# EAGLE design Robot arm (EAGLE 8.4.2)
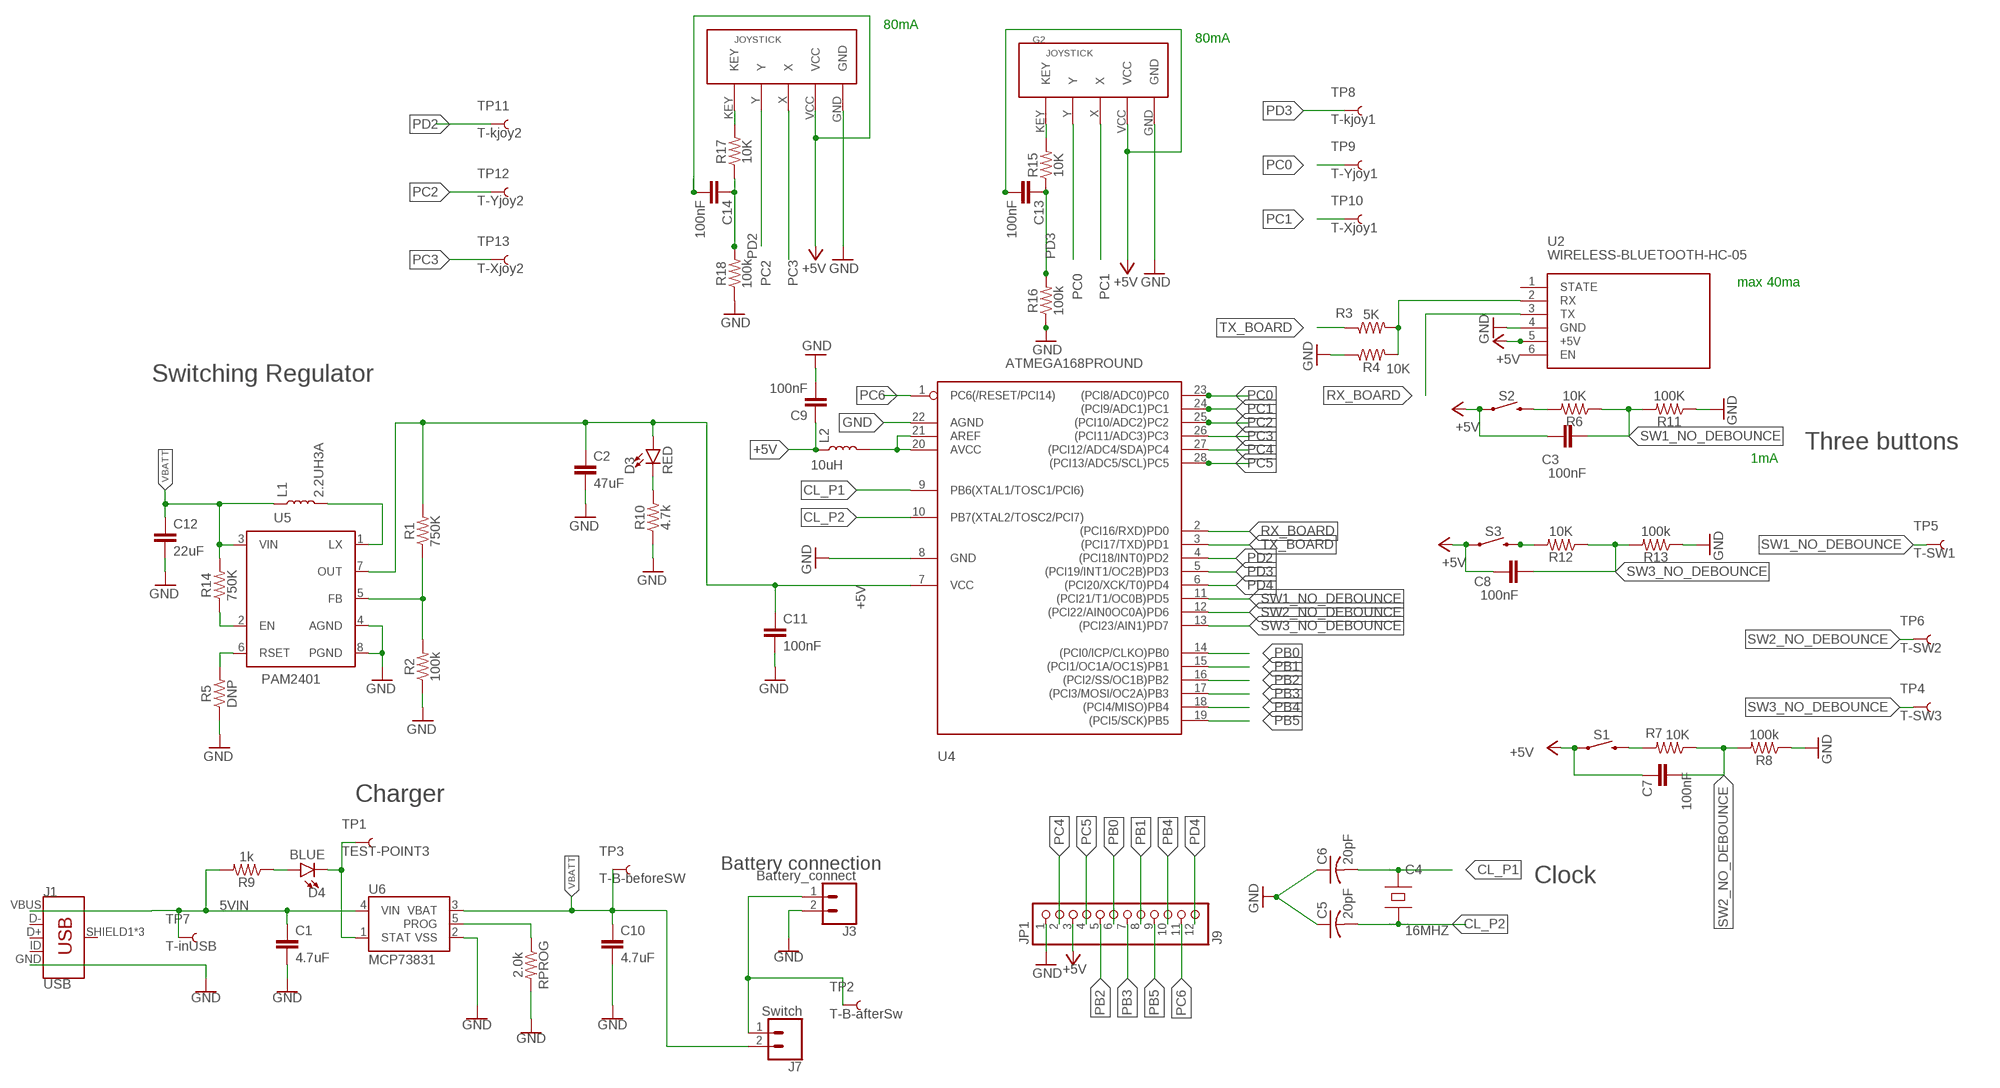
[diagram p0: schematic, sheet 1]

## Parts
C1  4.7uF  4.7UF0603  [0603]
C2  47uF  22UF-0805-6.3V-20%  [0805]
C3  100nF  10NF-0603-50V-10%  [0603]
C4  16MHZ  XTAL  [HC49UP]
C5  20pF  C-US025-025X050  [C025-025X050]
C6  20pF  C-US025-025X050  [C025-025X050]
C7  100nF  10NF-0603-50V-10%  [0603]
C8  100nF  10NF-0603-50V-10%  [0603]
C9  100nF  22UF-0805-6.3V-20%  [0805]
C10  4.7uF  4.7UF0603  [0603]
C11  100nF  22UF-0805-6.3V-20%  [0805]
C12  22uF  22UF-0805-6.3V-20%  [0805]
C13  100nF  10NF-0603-50V-10%  [0603]
C14  100nF  10NF-0603-50V-10%  [0603]
D3  RED  LED-RED0603  [LED-0603]
D4  BLUE  LED-BLUE0603  [LED-0603]
G1  G1  JOYSTICK  [JOYSTICK]
G2  G2  JOYSTICK  [JOYSTICK]
J1  USB  USB_MICRO-B_FEMALE-SMT  [USB-B-MICRO-SMD]
J3  Battery_connect  CONN_02  [1X02]
J7  Switch  CONN_02  [1X02]
JP1  J9  PINHD-1X12  [1X12]
L1  2.2UH3A  INDUCTOR-IFSC1515AHER2R2M01  [INDUCTOR_4X4MM]
L2  10uH  INDUCTOR-IFSC1515AHER2R2M01  [INDUCTOR_4X4MM]
R1  750K  750KOHM-0603-1/10W-1%  [0603]
R2  100k  100KOHM-0603-1/10W-1%  [0603]
R3  5K  10MOHM-0603-1/10W-5%  [0603]
R4  10K  10MOHM-0603-1/10W-5%  [0603]
R5  DNP  100KOHM-0603-1/10W-1%  [0603]
R6  10K  10MOHM-0603-1/10W-5%  [0603]
R7  10K  10MOHM-0603-1/10W-5%  [0603]
R8  100k  10MOHM-0603-1/10W-5%  [0603]
R9  1k  1KOHM-0603-1/10W-1%  [0603]
R10  4.7k  4.7KOHM-0603-1/10W-1%  [0603]
R11  100K  10MOHM-0603-1/10W-5%  [0603]
R12  10K  10MOHM-0603-1/10W-5%  [0603]
R13  100k  10MOHM-0603-1/10W-5%  [0603]
R14  750K  750KOHM-0603-1/10W-1%  [0603]
R15  10K  10MOHM-0603-1/10W-5%  [0603]
R16  100k  10MOHM-0603-1/10W-5%  [0603]
R17  10K  10MOHM-0603-1/10W-5%  [0603]
R18  100k  10MOHM-0603-1/10W-5%  [0603]
RPROG  2.0k  2.0KOHM-0603-1/10W-5%  [0603]
S1  MOMENTARY-SWITCH-SPST-SMD-6.2MM-TALL  [TACTILE_SWITCH_SMD_6.2MM_TALL]
S2  MOMENTARY-SWITCH-SPST-SMD-6.2MM-TALL  [TACTILE_SWITCH_SMD_6.2MM_TALL]
S3  MOMENTARY-SWITCH-SPST-SMD-6.2MM-TALL  [TACTILE_SWITCH_SMD_6.2MM_TALL]
TP1  TEST-POINT3  [PAD.03X.03]
TP2  T-B-afterSw  TEST-POINT3  [PAD.03X.03]
TP3  T-B-beforeSW  TEST-POINT3  [PAD.03X.03]
TP4  T-SW3  TEST-POINT3  [PAD.03X.03]
TP5  T-SW1  TEST-POINT3  [PAD.03X.03]
TP6  T-SW2  TEST-POINT3  [PAD.03X.03]
TP7  T-inUSB  TEST-POINT3  [PAD.03X.03]
TP8  T-kjoy1  TEST-POINT3  [PAD.03X.03]
TP9  T-Yjoy1  TEST-POINT3  [PAD.03X.03]
TP10  T-Xjoy1  TEST-POINT3  [PAD.03X.03]
TP11  T-kjoy2  TEST-POINT3  [PAD.03X.03]
TP12  T-Yjoy2  TEST-POINT3  [PAD.03X.03]
TP13  T-Xjoy2  TEST-POINT3  [PAD.03X.03]
U2  WIRELESS-BLUETOOTH-HC-05  [WIRELESS-BLUETOOTH-HC-05]
U4  ATMEGA168PROUND  [DIL28-3-ROUND]
U5  PAM2401  [MSOP8]
U6  MCP73831  [SOT23-5]

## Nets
5VIN: C1.1 J1.VBUS R9.2 TP7.P$1 U6.4(VIN)
+5V: C2.1 C3.1 C7.1 C8.1 C9.1 C11.1 C13.2 C14.2 D3.A G1.VCC G2.VCC JP1.3 L2.P$1 R1.2 S1.A2 S2.A2 S3.A2 U2.5(+5V) U4.7(VCC) U5.7(OUT)
AREF: L2.P$2 U4.20(AVCC) U4.21(AREF)
CL_P1: C4.1(A) C6.2 U4.9(PB6(XTAL1/TOSC1/PCI6))
CL_P2: C4.2(B) C5.2 U4.10(PB7(XTAL2/TOSC2/PCI7))
EN: R14.1 U5.2(EN)
GND: C1.2 C2.2 C5.1 C6.1 C9.2 C10.2 C11.2 C12.2 G1.GND G2.GND J1.GND J3.2 JP1.1 R2.1 R4.1 R5.1 R8.1 R10.1 R11.1 R13.1 R16.1 R18.1 RPROG.2 U2.4(GND) U4.8(GND) U4.22(AGND) U5.4(AGND) U5.8(PGND) U6.2(VSS)
N$2: D3.C R10.2
N$3: D4.A R9.1
N$4: L1.P$2 U5.1(LX)
N$5: G2.KEY R15.2
N$6: R5.2 U5.6(RSET)
N$7: G1.KEY R17.2
N$9: J3.1 J7.1 TP2.P$1
N$11: RPROG.1 U6.5(PROG)
N$12: R1.1 R2.2 U5.5(FB)
N$14: D4.C TP1.P$1 U6.1(STAT)
N$15: R7.2 S1.B2
N$16: R12.2 S3.B2
PB0: JP1.6 U4.14((PCI0/ICP/CLKO)PB0)
PB1: JP1.8 U4.15((PCI1/OC1A/OC1S)PB1)
PB2: JP1.5 U4.16((PCI2/SS/OC1B)PB2)
PB3: JP1.7 U4.17((PCI3/MOSI/OC2A)PB3)
PB4: JP1.10 U4.18((PCI4/MISO)PB4)
PB5: JP1.9 U4.19((PCI5/SCK)PB5)
PC0: G2.Y TP9.P$1 U4.23((PCI8/ADC0)PC0)
PC1: G2.X TP10.P$1 U4.24((PCI9/ADC1)PC1)
PC2: G1.Y TP12.P$1 U4.25((PCI10/ADC2)PC2)
PC3: G1.X TP13.P$1 U4.26((PCI11/ADC3)PC3)
PC4: JP1.2 U4.27((PCI12/ADC4/SDA)PC4)
PC5: JP1.4 U4.28((PCI13/ADC5/SCL)PC5)
PC6: JP1.11 U4.1(PC6(/RESET/PCI14))
PD2: C14.1 R17.1 R18.2 TP11.P$1 U4.4((PCI18/INT0)PD2)
PD3: C13.1 R15.1 R16.2 TP8.P$1 U4.5((PCI19/INT1/OC2B)PD3)
PD4: JP1.12 U4.6((PCI20/XCK/T0)PD4)
RX: R3.2 R4.2 U2.2(RX)
RX_BOARD: U2.3(TX) U4.2((PCI16/RXD)PD0)
SW1_BOUNCE: R6.2 S2.B2
SW1_NO_DEBOUNCE: C3.2 R6.1 R11.2 TP5.P$1 U4.11((PCI21/T1/OC0B)PD5)
SW2_NO_DEBOUNCE: C7.2 R7.1 R8.2 TP6.P$1 U4.12((PCI22/AIN0OC0A)PD6)
SW3_NO_DEBOUNCE: C8.2 R12.1 R13.2 TP4.P$1 U4.13((PCI23/AIN1)PD7)
TX_BOARD: R3.1 U4.3((PCI17/TXD)PD1)
VBATT: C10.1 C12.1 J7.2 L1.P$1 R14.2 TP3.P$1 U5.3(VIN) U6.3(VBAT)
Unconnected: J1.D+ J1.D- J1.ID J1.SHIELD1(SHIELD) J1.SHIELD2(SHIELD) J1.SHIELD3(SHIELD) U2.1(STATE) U2.6(EN)

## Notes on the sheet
- 80mA
- 80mA
- max 40ma
- Switching Regulator
- Three buttons
- 1mA
- Charger
- Battery connection
- Clock

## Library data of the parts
C1 C10 = SparkFun-Capacitors:4.7UF: 4.7µF ceramic capacitors; PROD_ID: CAP-08280
C2 C9 C11 = SparkFun-Capacitors:22UF: 22µF ceramic capacitors; PROD_ID: CAP-08402; VALUE: 22uF
C3 C7 C8 C13 C14 = SparkFun-Capacitors:10NF: 0.01uF/10nF/10,000pF ceramic capacitors; PROD_ID: CAP-00867; VALUE: 10nF
C4 = Misc:XTAL: Piezoelectric crystal. Set C, Lser and Cpar to set series and parallel resonances. This is actually the same as a capacitor.
C5 C6 = adafruit:C-US: CAPACITOR, American symbol
C12 = SparkFun-Capacitors:22UF: 22µF ceramic capacitors; PROD_ID: CAP-08402
D3 = SparkFun-LED:LED-RED: Red SMD LED; PROD_ID: DIO-00819
D4 = SparkFun-LED:LED-BLUE: Blue SMD LED; PROD_ID: DIO-08575
G1 G2 = joystick:JOYSTICK
J1 = SparkFun-Connectors:USB_MICRO-B: USB Type Micro-B Connector Male/female and PTH/SMT variants SparkFun Products: SparkFun microB USB Breakout SparkFun USB microB Plug Breakout SparkFun ESP8266 Thing; PROD_ID: CONN-11752
J3 J7 = SparkFun-Connectors:CONN_02: Multi connection point. Often used as Generic Header-pin footprint for 0.1 inch spaced/style header connections
JP1 = adafruit:PINHD-1X12: PIN HEADER
L1 = SparkFun-Coils:INDUCTOR: Inductors; PROD_ID: NDUC-13770
L2 = SparkFun-Coils:INDUCTOR: Inductors; PROD_ID: NDUC-13770; VALUE: 2.2UH3A
R1 R14 = SparkFun-Resistors:750KOHM: 750Ω resistor; PROD_ID: RES-13768
R2 = SparkFun-Resistors:100KOHM: 100kΩ resistor; PROD_ID: RES-07828
R3 R4 R6-R8 R11-R13 R15-R18 = SparkFun-Resistors:10MOHM: RES-09327; PROD_ID: RES-08283; VALUE: 10M
R5 = SparkFun-Resistors:100KOHM: 100kΩ resistor; PROD_ID: RES-07828; VALUE: 100k
R9 = SparkFun-Resistors:1KOHM: 1kΩ resistor; PROD_ID: RES-07856
R10 = SparkFun-Resistors:4.7KOHM: 4.7kΩ resistor; PROD_ID: RES-07857
RPROG = SparkFun-Resistors:2.0KOHM: 2kΩ resistor; PROD_ID: RES-08296
S1-S3 = SparkFun-Switches:MOMENTARY-SWITCH-SPST: Momentary Switch (Pushbutton) - SPST; PROD_ID: SWCH-11966; SF_SKU: COM-12992
TP1-TP13 = SparkFun-Connectors:TEST-POINT: SparkFun Test Points
U2 = diy-modules:WIRELESS-BLUETOOTH-HC-05: Bluetooth Transceiver Module based on HC-05 board Tutorial is available here: https://arduino-info.wikispaces.com/BlueTooth-HC05-HC06-Modules-How-To Click here to find device on ebay.com
U4 = adafruit:ATMEGA168*P: MICROCONTROLLER 16 kBytes FLASH 1 kBytes SRAM 512 Bytes EEPROM USART 8-channel 10 bit ADC
U5 = SparkFun-IC-Power:PAM2401: PAM2401 - Boost PMIC Specifications: Up to 1A output current 0.9V to 4.75V Input Range 2.5V to 5.0V Adjustable Output Voltage Datasheet (Diodes inc.); PROD_ID: IC-13769
U6 = SparkFun-IC-Power:MCP73831: MCP73831T Li-Ion, Li-Pol Controller Miniature single cell, fully integrated Li-Ion, Li-polymer charge management controller Datasheet SparkFun Products: SparkFun ESP32 Thing SparkFun 9DoF Razor IMU M0; PROD_ID: IC-09995

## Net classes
0 default: width 0.152 mm, drill 0.305 mm, clearance 0.152 mm
1 +5V: width 117 mm
2 GND: width 117 mm

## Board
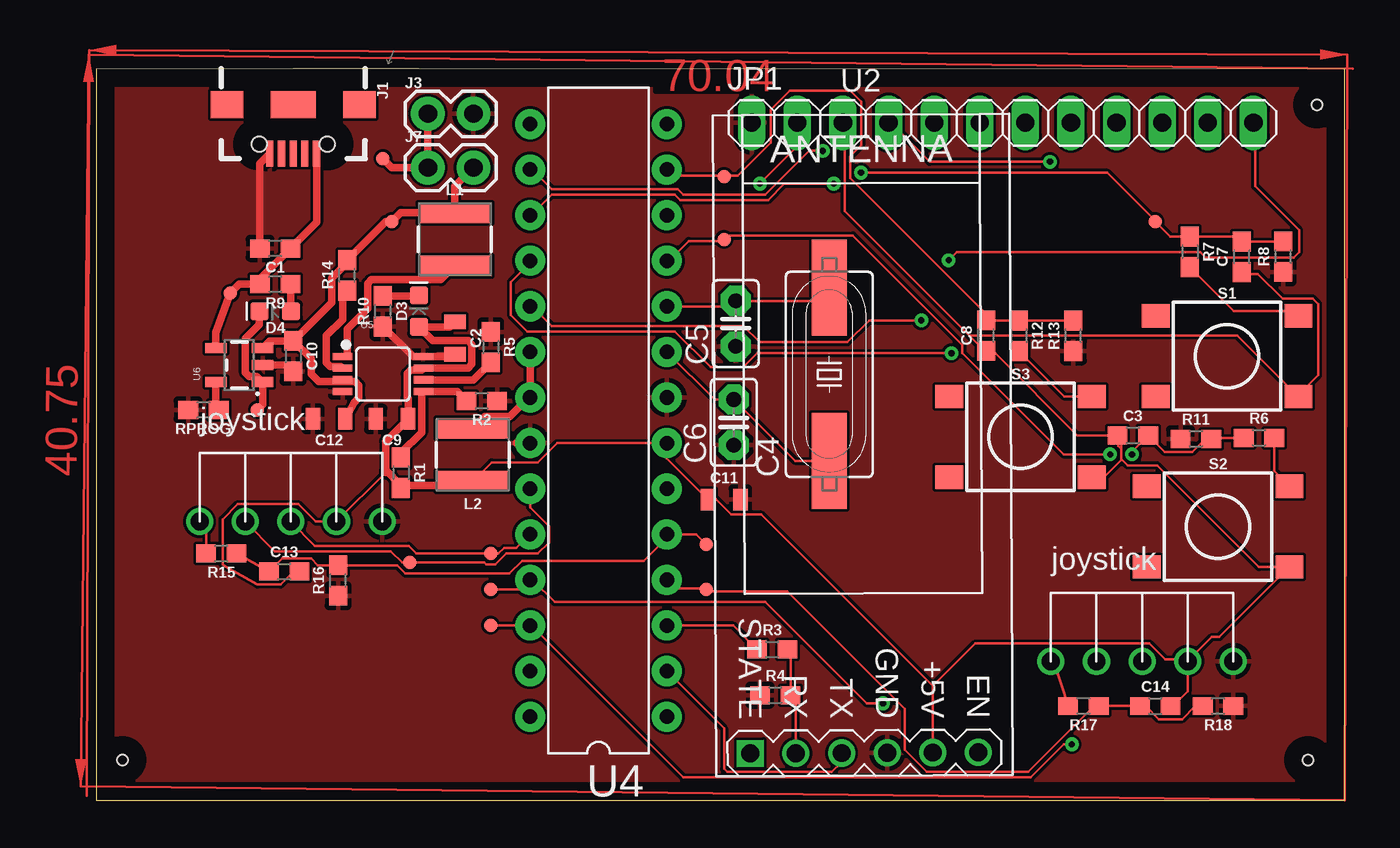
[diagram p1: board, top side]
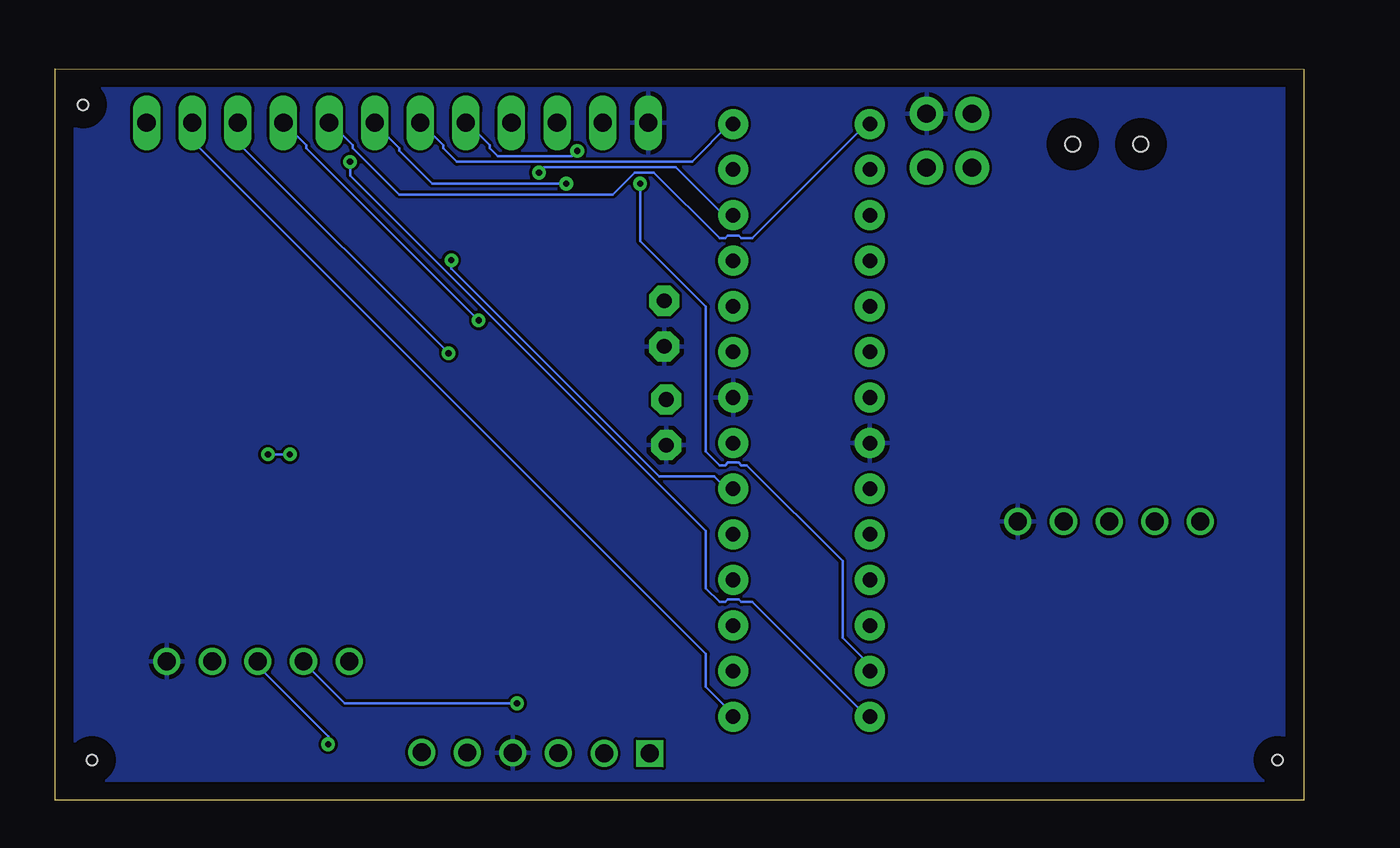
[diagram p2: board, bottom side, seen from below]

Size 69.51 x 40.76 mm. Coordinates in mm from the lower left corner, seen from the top.
Outline: 0,0 69.51,0.01 69.51,40.76 0,40.75 0,0
Copper layers (1*16): Top 0.035mm / dielectric 1.5mm / Bottom 0.035mm
Design rules "default": minimum track width 6mil, minimum drill 0.35mm, track to track 6mil, track to pad 6mil, pad to pad 6mil, via to via 6mil, smd to smd 6mil, copper to edge 40mil, drill to drill 6mil, minimum pad ring 10mil, minimum via ring 8mil, stop-mask expansion 4mil, vias tented up to drill 0mil, thermal gap 10mil
Holes 0.6 mm at 67.97,38.76 1.47,2.26 67.47,2.26

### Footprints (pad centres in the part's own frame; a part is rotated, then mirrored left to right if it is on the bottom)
0603 = smd 1.1 x 1: 1 -0.85,0; 2 0.85,0
0805 = smd 0.8 x 1.2: 1 -0.9,0; 2 0.9,0
HC49UP = smd 5.334 x 1.93: 1 -4.826,0; 2 4.826,0
C025-025X050 = drill 0.813 pad 1.676 octagon: 1 -1.27,0; 2 1.27,0
LED-0603 = smd 1 x 1: A -0.877,0; C 0.877,0
JOYSTICK = drill 1: GND 6.35,0; KEY -3.81,0; VCC 3.81,0; X 1.27,0; Y -1.27,0
USB-B-MICRO-SMD = smd 1.45 x 0.4: D+ 2.725,0; D- 2.725,0.65; GND 2.725,-1.3; ID 2.725,-0.65; VBUS 2.725,1.3 | smd 1.5 x 1.8: SHIELD1 0,3.685; SHIELD2 0,-3.685 | smd 1.5 x 2.5: SHIELD3 0,0 | hole 0.85: 2.2,1.9; 2.2,-1.9
1X02 = drill 1.016 pad 1.88: 1 0,0; 2 2.54,0
1X12 = drill 1.016 long: 1 -13.97,0; 2 -11.43,0; 3 -8.89,0; 4 -6.35,0; 5 -3.81,0; 6 -1.27,0; 7 1.27,0; 8 3.81,0; 9 6.35,0; 10 8.89,0; 11 11.43,0; 12 13.97,0
INDUCTOR_4X4MM = smd 4.089 x 1.143: P$1 0,1.473; P$2 0,-1.473
TACTILE_SWITCH_SMD_6.2MM_TALL = smd 1.55 x 1.3: A1 -3.975,-2.25; A2 3.975,-2.25; B1 -3.975,2.25; B2 3.975,2.25
PAD.03X.03 = smd 0.762 x 0.762: P$1 0,0
WIRELESS-BLUETOOTH-HC-05 = drill 1 square: 1 -6.35,-17.145 | drill 1: 2 -3.81,-17.145; 3 -1.27,-17.145; 4 1.27,-17.145; 5 3.81,-17.145; 6 6.35,-17.145
DIL28-3-ROUND = drill 0.813 pad 1.676: 1 -16.51,-3.81; 2 -13.97,-3.81; 3 -11.43,-3.81; 4 -8.89,-3.81; 5 -6.35,-3.81; 6 -3.81,-3.81; 7 -1.27,-3.81; 8 1.27,-3.81; 9 3.81,-3.81; 10 6.35,-3.81; 11 8.89,-3.81; 12 11.43,-3.81; 13 13.97,-3.81; 14 16.51,-3.81; 15 16.51,3.81; 16 13.97,3.81; 17 11.43,3.81; 18 8.89,3.81; 19 6.35,3.81; 20 3.81,3.81; 21 1.27,3.81; 22 -1.27,3.81; 23 -3.81,3.81; 24 -6.35,3.81; 25 -8.89,3.81; 26 -11.43,3.81; 27 -13.97,3.81; 28 -16.51,3.81
MSOP8 = smd 0.4 x 1.1: 1 -0.975,-2.25; 2 -0.325,-2.25; 3 0.325,-2.25; 4 0.975,-2.25; 5 0.975,2.25; 6 0.325,2.25; 7 -0.325,2.25; 8 -0.975,2.25
SOT23-5 = smd 0.55 x 1.2: 1 -0.95,-1.3; 2 0,-1.3; 3 0.95,-1.3; 4 0.95,1.3; 5 -0.95,1.3

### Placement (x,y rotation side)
C1  9.97,30.76 180 top
C2  19.97,25.76 270 top
C3  57.73,20.34 0 top
C4  40.82,23.74 90 top
C5  35.62,26.57 90 top
C6  35.51,21.07 90 top
C7  63.8,30.29 90 top
C8  49.56,25.9 90 top
C9  16.47,21.26 180 top
C10  10.97,24.76 270 top
C11  34.97,16.76 0 top
C12  12.97,21.26 180 top
C13  10.47,12.76 0 top
C14  58.97,5.26 0 top
D3  17.97,27.26 90 top
D4  9.97,27.26 180 top
G1  56.97,7.76 0 top
G2  9.57,15.54 0 top
J1  10.97,38.76 270 top
J3  18.47,38.26 0 top
J7  18.47,35.26 0 top
JP1  50.47,37.76 0 top
L1  19.97,31.26 0 top
L2  20.97,19.26 180 top
R1  16.97,18.26 270 top
R2  21.47,22.26 180 top
R3  37.65,8.41 0 top
R4  37.82,5.87 0 top
R5  21.97,25.26 270 top
R6  64.75,20.21 0 top
R7  60.91,30.56 270 top
R8  66.1,30.3 90 top
R9  9.97,28.76 180 top
R10  15.97,27.26 90 top
R11  61.24,20.15 0 top
R12  51.37,25.89 270 top
R13  54.42,25.88 90 top
R14  13.97,29.26 90 top
R15  6.97,13.76 180 top
R16  13.47,12.26 90 top
R17  54.97,5.26 180 top
R18  62.47,5.26 180 top
RPROG  5.97,21.76 180 top
S1  62.97,24.76 0 top
S2  62.47,15.26 0 top
S3  51.47,20.26 0 top
TP1  8.97,21.76 0 top
TP2  15.97,35.76 0 top
TP3  16.47,32.26 0 top
TP4  34.97,34.76 0 top
TP5  34.97,31.26 0 top
TP6  58.97,32.26 0 top
TP7  7.47,28.26 0 top
TP8  33.97,14.26 0 top
TP9  17.47,13.26 0 top
TP10  21.97,13.76 0 top
TP11  33.97,11.76 0 top
TP12  21.97,11.76 0 top
TP13  21.97,9.76 0 top
U2  42.69,19.79 0.3 top
U4  27.97,21.18 90 top
U5  15.97,23.76 270 top
U6  7.97,24.26 90 top

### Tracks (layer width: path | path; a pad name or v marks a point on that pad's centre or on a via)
5VIN
  Top 0.406: U6.4 6.67,26.06 TP7.P$1 7.97,28.76 R9.2 9.12,29.06 C1.1 12.27,32.21 J1.VBUS
+5V
  Top 0.152: 34.02,16.81 C11.1 | 34.02,16.81 31.78,19.05 U4.7 25.67,19.91 24.61,18.84 22.03,18.84 L2.P$1 | 59.97,5.26 60.25,5.26 | C14.2 59.97,5.26 | C7.1 63.93,29.34 64.7,29.34 66.07,27.97 67.74,27.97 68.05,27.66 68.05,23.7 66.98,22.63 S1.A2 63.55,25.91 48.62,25.91 | C3.1 56.92,20.19 56.92,19.74 57.08,19.58 57.08,18.98 56.16,18.06 55.55,18.06 S3.A2 | C3.1 56.77,20.35 54.64,20.35 50.06,24.92 49.61,24.92 C8.1 49.45,25.07 48.62,25.91 | 48.62,25.91 41.68,32.84 41.68,37.72 JP1.3 | 59.97,5.26 60.78,6.07 G1.VCC 60.88,7.85 | 60.88,7.85 62.13,9.1 62.54,9.1 S2.A2 64.75,13.01 59.08,18.67 57.43,18.67 57.08,19.03 57.08,20.14 C3.1 | U2.5 46.59,6.37 | 46.59,6.37 37.03,15.93 35.38,15.93 34.5,16.81 34.02,16.81 | 60.88,7.85 59.54,7.85 58.65,8.74 48.96,8.74 46.59,6.37 | C13.2 11,12.76 10.27,12.03 8.98,12.03 7.18,13.03 7.04,13.16 7.04,15.67 7.9,16.52 11.25,16.52 12.23,15.54 G2.VCC 16.12,18.28 16.12,18.41
  Top 0.406: 16.97,17.55 R1.2 | 16.12,18.41 16.97,17.55 | 16.12,18.41 16.12,20 C9.1 17.37,22.38 17.32,22.44 17.32,23.78 17.53,23.99 18.13,23.99 U5.7 18.24,24.1 20.72,24.1 20.93,24.31 20.93,25.41 20.72,25.61 18.74,25.61 D3.A 19.7,26.38 C2.1 | L2.P$1 19.74,17.55 16.97,17.55 | 16.12,18.27 16.12,18.41
AREF
  Top 0.406: U4.20 U4.21 24.07,22.45 23.02,21.4 21.64,21.4 L2.P$2
CL_P1
  Top 0.152: U4.9 34.44,22.34 C6.2 38.93,18.91 C4.1
CL_P2
  Top 0.152: U4.10 35.31,27.53 C5.2 40.09,27.84 C4.2
EN
  Top 0.406: R14.1 13.72,28.16 13.72,26.8 12.82,25.89 12.82,24.39 13.03,24.17 13.63,24.17 U5.2
GND
  Top 0.406: C10.2 10.62,24.26 U6.2 | U4.22 23.39,19.91 | C2.2 19.85,24.73 U5.8 17.65,24.73 R10.1 | J1.GND 9.12,35.48 C1.2
  pour Top: -15.37,-9.52 79.63,-10.29 78.11,41.78 -15.62,41.53
  pour Bottom: -17.14,-11.3 80.65,-11.56 80.39,43.31 -17.4,43.56
N$2
  Top 0.406: R10.2 17.95,28.11 D3.C
N$3
  Top 0.406: D4.A 10.85,28.73 R9.1
N$4
  Top 0.406: L1.P$2 19.2,29.01 15.33,29.01 15.12,28.8 15.12,27.4 13.97,26.26 13.97,24.76 13.95,24.73 U5.1
N$5
  Top 0.152: G2.KEY 6.12,15.18 R15.2
N$6
  Top 0.406: R5.2 21,23.43 U5.6
N$7
  Top 0.152: R17.2 53.32,7.76 G1.KEY
N$9
  Top 0.406: TP2.P$1 16.47,35.26 J7.1 J3.1
N$11
  Top 0.406: RPROG.1 6.67,21.91 U6.5
N$12
  Top 0.406: R1.1 16.97,19.36 18.13,20.51 18.13,22.69 U5.5 20.1,22.78 R2.2
N$14
  Top 0.406: TP1.P$1 9.27,22.06 U6.1 8.96,23.63 8.53,23.63 8.32,23.84 8.32,25.73 9.1,26.5 D4.C
N$15
  Top 0.152: R7.2 63.36,27.26 66.47,27.26 66.72,27.01 S1.B2
N$16
  Top 0.152: R12.2 53.9,22.51 S3.B2
PB0
  Bottom 0.152: JP1.6 49.15,37.72 47.93,36.5 47.93,36.35 47.17,35.59 34.06,35.59 31.93,37.72 U4.14
PB1
  Bottom 0.152: JP1.8 54.18,37.72 52.96,36.5 52.96,36.35 50.37,33.76 38.48,33.76 37.26,34.98 36.2,34.98 32.54,31.32 32.23,31.32 32.08,31.47 31.47,31.47 31.32,31.32 30.71,31.32 24.31,37.72 U4.15
PB2  (via drill 0.35)
  Top 0.152: v40.46,36.2 39.7,36.2 37.26,33.76 32.69,33.76 32.39,34.06 25.38,34.06 24.31,35.13 U4.16
  Bottom 0.152: v40.46,36.2 40.77,35.89 44.88,35.89 45.34,36.35 45.34,36.5 46.56,37.72 JP1.5
PB3  (via drill 0.35)
  Top 0.152: v41.07,34.37 38.33,34.37 37.42,33.45 32.54,33.45 32.23,33.76 25.38,33.76 24.31,32.69 U4.17
  Bottom 0.152: v41.07,34.37 48.54,34.37 50.37,36.2 50.37,36.35 51.74,37.72 JP1.7
PB4  (via drill 0.35)
  Top 0.152: v47.63,24.92 36.81,24.92 36.04,24.16 34.22,24.16 32.23,26.14 24,26.14 23.09,27.05 23.09,28.88 24.16,29.95 U4.18
  Bottom 0.152: v47.63,24.92 59.36,36.65 59.36,37.72 JP1.10
PB5  (via drill 0.35)
  Top 0.152: v45.95,26.75 43.05,26.75 41.84,25.53 36.96,25.53 36.04,26.44 25.38,26.44 24.31,27.51 U4.19
  Bottom 0.152: v45.95,26.75 55.55,36.35 55.55,36.5 56.77,37.72 JP1.9
PC0
  Top 0.152: TP9.P$1 17.9,13.26 | TP9.P$1 21.61,13.26 21.72,13.15 22.23,13.15 22.84,13.76 24.61,13.76 25.23,14.39 25.23,15.27 24.16,16.34 U4.23 | TP9.P$1 17.04,13.26 16.41,13.89 9.95,13.89 G2.Y
PC1
  Top 0.152: U4.24 23.4,14.07 22.71,14.07 22.4,13.76 TP10.P$1 17.84,13.76 17.4,14.19 12.19,14.19 G2.X
PC2  (via drill 0.35)
  Top 0.152: TP12.P$1 23.63,11.76 U4.25 24.31,12.27 25.53,11.05 37.26,11.05 42.9,5.41 v43.82,5.41
  Bottom 0.152: 55.37,7.36 55.33,7.33 55.33,7.17 | 55.37,7.36 55.64,7.63 G1.Y | v43.82,5.41 53.42,5.41 55.37,7.36
PC3  (via drill 0.35)
  Top 0.152: TP13.P$1 U4.26 24.31,9.68 32.69,1.3 52.05,1.3 53.87,3.12 v54.33,3.12
  Bottom 0.152: v54.33,3.12 54.33,3.58 57.92,7.17 57.92,7.33 58.23,7.63 G1.X
PC4  (via drill 0.35)
  Top 0.152: v36.96,34.37 38.94,36.35 38.94,37.72 JP1.2
  Bottom 0.152: v36.96,34.37 36.96,31.17 33.3,27.51 33.3,19.43 32.54,18.67 32.23,18.67 32.08,18.82 31.47,18.82 31.32,18.67 31.01,18.67 25.68,13.34 25.68,9.07 24.31,7.7 24.31,7.24 U4.27
PC5  (via drill 0.35)
  Top 0.152: v53.11,35.59 46.41,35.59 44.27,37.72 JP1.4
  Bottom 0.152: v53.11,35.59 53.11,34.82 33.3,15.01 33.3,11.81 32.54,11.05 32.23,11.05 32.08,11.2 31.47,11.2 31.32,11.05 30.71,11.05 24.31,4.65 U4.28
PC6
  Bottom 0.152: JP1.11 61.8,37.72 61.8,36.65 33.3,8.15 33.3,6.33 31.78,4.8 U4.1
PD2
  Top 0.152: C14.1 R17.1 55.79,5.19 55.48,5.19 51.89,1.6 46.25,1.6 45.04,2.82 45.04,5.11 38.48,11.66 34.06,11.66 TP11.P$1 33.91,11.81 32.39,11.81 31.93,12.27 U4.4 | C14.1 58.45,5.26 | 61.2,5.26 R18.2 61.2,5.26 | C14.1 58.45,5.26 | 58.45,5.26 59.18,4.53 60.47,4.53 61.2,5.26
PD3
  Top 0.152: 31.97,14.83 33.4,14.83 TP8.P$1 | R15.1 C13.1 10.35,13.49 11.97,13.49 12.35,13.11 R16.2 16.76,13.11 17.22,12.65 23.02,12.65 23.72,13.36 30.5,13.36 31.97,14.83 | U4.5 31.97,14.83
PD4  (via drill 0.35)
  Top 0.152: v47.47,30.1 47.93,30.56 61.49,30.56 61.8,30.25 66.68,30.25 66.98,30.56 66.98,31.78 64.54,34.21 64.54,37.72 JP1.12
  Bottom 0.152: v47.47,30.1 47.47,29.64 35.89,18.06 32.84,18.06 32.23,17.45 31.93,17.45 U4.6
RX
  Top 0.152: U2.2 38.97,5.56 R4.2 38.67,8.25 R3.2
RX_BOARD
  Top 0.152: U4.2 34.97,4.02 34.97,1.76 35.13,1.6 40.97,1.6 41.51,2.14 U2.3
SW1_BOUNCE
  Top 0.152: R6.2 65.6,18.35 S2.B2
SW1_NO_DEBOUNCE  (via drill 0.35)
  Top 0.152: R6.1 62.14,20.21 R11.2 61.76,20.15 61.03,19.42 59.5,19.42 C3.2 58.45,20.19 57.68,19.43 v57.68,19.28 | U4.11 31.93,30.1 33,31.17 34.82,31.17 TP5.P$1 34.98,31.32 35.13,31.47 42.14,31.47 48.24,25.38 48.24,24.92 53.87,19.28 v56.47,19.28
  Bottom 0.152: v56.47,19.28 v57.68,19.28
SW2_NO_DEBOUNCE  (via drill 0.35)
  Top 0.152: R8.2 C7.2 63.53,31.41 R7.1 59.82,31.41 TP6.P$1 58.9,32.39 56.31,34.98 v42.6,34.98
  Bottom 0.152: v42.6,34.98 42.29,35.28 34.98,35.28 32.39,32.69 31.93,32.69 U4.12
SW3_NO_DEBOUNCE
  Top 0.152: R13.2 R12.1 51.36,26.75 C8.2 49.45,26.9 49.45,27.2 41.99,34.67 41.99,35.89 42.6,36.5 42.6,38.94 41.99,39.55 38.63,39.55 37.57,38.48 37.57,36.65 35.74,34.82 34.98,34.82 TP4.P$1 34.82,34.82 32.23,34.82 31.93,35.13 U4.13
TX_BOARD
  Top 0.152: R3.1 35.47,9.75 U4.3
VBATT
  Top 0.406: U6.3 9.67,25.61 C10.1 | J7.2 19.97,34.22 L1.P$1 19.5,32.73 19.47,32.76 16.97,32.76 TP3.P$1 16.12,32.26 R14.2 13.87,30.01 13.87,29.86 13.12,29.1 13.12,27.75 C10.1 | 13.82,23.34 14.42,23.34 14.63,23.13 14.63,22.44 14.37,22.18 C12.1 | U5.3 13.82,23.34 | C10.1 11.97,24.61 11.97,23.76 12.39,23.34 13.82,23.34
(copper drawn outside any net)
  shapes: Top area x4

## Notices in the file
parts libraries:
diy-modules: Released under the Creative Commons Attribution 4.0 International License: http://creativecommons.org/licenses/by/4.0
SparkFun-Capacitors: Licensing: CC v3.0 Share-Alike You are welcome to use this library for commercial purposes.
